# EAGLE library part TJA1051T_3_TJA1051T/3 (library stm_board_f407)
High-speed CAN transceiver The TJA1051 is a high-speed CAN transceiver that provides an interface between a Controller Area Network (CAN) protocol controller and the physical two-wire CAN bus. The transceiver is designed for high-speed (up to 1 Mbit/s) CAN applications in the automotive industry, providing differential transmit and receive capability to (a microcontroller with) a CAN protocol controller. The TJA1051 belongs to the third generation of high-speed CAN transceivers from NXP Semiconductors, offering significant improvements over first- and second-generation devices such as the TJA1050. It offers improved ElectroMagnetic Compatibility (EMC) and ElectroStatic Discharge (ESD) performance, and also features: Ideal passive behavior to the CAN bus when the supply voltage is off TJA1051T/3 and TJA1051TK/3 can be interfaced directly to microcontrollers with supply voltages from 3 V to 5 V These features make the TJA1051 an excellent choice for all types of HS-CAN networks, in nodes that do not require a standby mode with wake-up capability via the bus. AAL Eindhoven MK Check prices
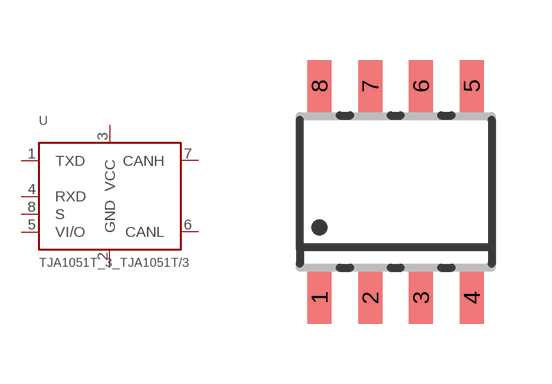
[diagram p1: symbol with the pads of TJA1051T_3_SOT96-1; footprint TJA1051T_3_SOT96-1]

Designator prefix U

## TJA1051T_3_TJA1051T/3 (AVAILABILITY: Bad; DESCRIPTION: 1/1 Transceiver Half CANbus 8-SO; MF: NXP Semiconductors; MP: TJA1051T/3; PACKAGE: SOIC-8 NXP Semiconductors; PRICE: None)  [TJA1051T_3_SOT96-1]
1  TXD  out
2  GND
3  VCC
4  RXD
5  VI/O  pas
6  CANL
7  CANH
8  S  pwr

## Footprint TJA1051T_3_SOT96-1 (pad centres in mm)
SOT96-1 SO8: plastic small outline package; 8 leads; body width 3.9 mm JEDEC: MS-012 IEC: 076E03
smd 0.6 x 1.3: 1 -1.905,-2.65; 2 -0.635,-2.65; 3 0.635,-2.65; 4 1.905,-2.65; 5 1.905,2.65; 6 0.635,2.65; 7 -0.635,2.65; 8 -1.905,2.65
